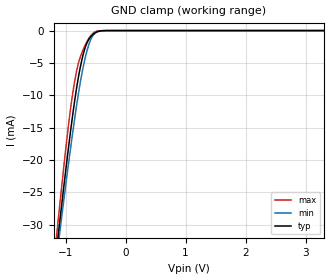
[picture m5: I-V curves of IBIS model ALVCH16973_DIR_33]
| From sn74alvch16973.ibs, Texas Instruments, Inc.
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[Model]   ALVCH16973_DIR_33
Model_type  Input
Vinl=0.8
Vinh=2.0
| variable   typ   min   max
C_comp   2.48pF   2.02pF   3.12pF
[Temperature Range]   40   100   -40
| Ambient temperature   25   85   -40
[Voltage range]   3.3   3   3.6
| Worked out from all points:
|   GND clamp passes 1 mA (typ) near -0.58 V on its own axis
[GND Clamp]
| ALVCH16973_DIR_33
|   Voltage   I(typ)   I(min)   I(max)
-3.3V     -229.2mA   -214.9mA   -246.1mA
-1.15V    -33.88mA   -35.24mA   -31.79mA
-1.125V   -31.83mA   -33.35mA   -29.52mA
-1.1V     -29.79mA   -31.47mA   -27.27mA
-1.075V   -27.77mA   -29.61mA   -25.05mA
-940mV    -17.28mA   -19.83mA   -13.78mA
-825mV    -9.422mA   -12.15mA   -6.674mA
-750mV    -5.474mA   -7.789mA   -3.976mA
-675mV    -2.681mA   -4.31mA    -2.304mA
-590mV    -1.072mA   -1.6mA     -901.9uA
-515mV    -393.5uA   -457.8uA   -227.6uA
3.3V      193.8pA    964pA      46.32pA
